| TEXAS INSTRUMENTS INCORPORATED
| Standard Linear and Logic Group
| IBIS Model of SN74AVCH16T245
| 16-Bit Dual-Supply Bus Transeiver with Configurable Voltage Translation and
| 3-State Outputs
| This file contains package information for the following:
|  TSSOP 48-pin (DGG) package as [Component] AVCH16T245_DGG
|  TVSOP 48-pin (DGV) package as [Component] AVCH16T245_DGV
|  U*BGA 48-pin (GQL) package as [Component] AVCH16T245_GQL
|  U*BGA 48-pin (ZQL) package as [Component] AVCH16T245_ZQL
| This device can be powered at the following Vccs:
|  1.2 volt Vcc
|  1.5 volt Vcc
|  1.8 volt Vcc
|  2.5 volt Vcc
|  3.3 volt Vcc
| This file provides unique models under the [Model Selector] for each Vcc.
| For operation at a specific Vcc, select the appropriate model after each
| [Model Selector] keyword.
[IBIS Ver]   3.2
[Comment char]  |_char
[File Name]   sn74avch16t245.ibs
[File Rev]   1.1 | x_die
[Date]   May 14, 2004
[Source]   Data created from TI-SPICE simulations at TI-SLL.
[Notes]   The following is an IBIS list for the AVCH16T245.
   Please contact sllibis@ti.com with questions and
   comments concerning SLL IBIS models.
   - FILE REV HISTORY
   - 1.1 Release IBIS file on 06/03/04
   - Power clamp data deleted as there is no power-clamp diode.
   - Non-monotonic data in ground-clamp due to bus-hold
   - Due to the fact that the Device is 4.6-V Input/Output
   tolarent, the I/O models has some Non-Monotonic Warnings.
[Disclaimer] Property of Texas Instruments Incorporated.  Unauthorized
   reproduction and/or distribution is strictly prohibited.
   This product is protected under copyright law.
   Created  2003, (C) Copyright  2003, Texas Instruments
   Incorporated, All Rights Reserved
   UNLESS THERE IS A SIGNED, WRITTEN AGREEMENT TO THE
   CONTRARY, TEXAS INSTRUMENTS (TI) IS PROVIDING THE IBIS
   MODELS  AND WITHOUT ANY WARRANTY, EXPRESSED OR
   IMPLIED.  TI assumes no liability for:
   1) the accuracy of the IBIS models provided to your
   company;
   2) the proper functioning of these IBIS Models in your
   design or for any resulting applications; or
   3) infringement of patents, copyrights or intellectual
   property rights resulting from your use of these IBIS
   models.
   TI provides IBIS Models as a service to our customers.
   You and your company shall not distribute, sell or give
   these models to anyone else without prior written
   permission from TI.
   TI reserves the right to make changes to our products or
   to discontinue any semiconductor product or service
   without notice, and advises our customers to obtain the
   latest version of relevant information to verify, before
   placing orders, that the information being relied on is
   current.
   Please be aware that your receipt and use of the IBIS
   information provided shall serve as acceptance of these
   terms and conditions.  If you do not accept these terms,
   you should return or destroy the IBIS models and any
   other accompanying information immediately.
| Component AVCH16T245_DGG 48-pin TSSOP
[Component]   AVCH16T245_DGG
[Manufacturer]   Texas Instruments, Inc.
[Package]
|   typ   min   max
R_pkg   6.200e-02   5.000e-02   7.800e-02
L_pkg   3.527e-09   3.128e-09   4.255e-09
C_pkg   5.300e-13   4.170e-13   6.850e-13
[Pin]   signal_name   model_name   R_pin   L_pin   C_pin
1   1DIR   AVCH16T245_DIR   5.000e-02   4.250e-09   6.710e-13
2   1b1   AVCH16T245_IO   5.700e-02   3.956e-09   6.740e-13
3   1b2   AVCH16T245_IO   7.100e-02   3.922e-09   6.190e-13
4   GND   GND   7.800e-02   3.841e-09   6.180e-13
5   1b3   AVCH16T245_IO   5.600e-02   3.535e-09   5.550e-13
6   1b4   AVCH16T245_IO   5.800e-02   3.464e-09   5.030e-13
7   VCCB   POWER   6.000e-02   3.362e-09   4.980e-13
8   1b5   AVCH16T245_IO   6.100e-02   3.293e-09   4.620e-13
9   1b6   AVCH16T245_IO   6.300e-02   3.240e-09   4.550e-13
10   GND   GND   6.300e-02   3.175e-09   4.420e-13
11   1b7   AVCH16T245_IO   6.400e-02   3.153e-09   4.290e-13
12   1b8   AVCH16T245_IO   6.500e-02   3.128e-09   4.180e-13
13   2b1   AVCH16T245_IO   6.500e-02   3.128e-09   4.180e-13
14   2b2   AVCH16T245_IO   6.400e-02   3.154e-09   4.290e-13
15   GND   GND   6.300e-02   3.174e-09   4.420e-13
16   2b3   AVCH16T245_IO   6.300e-02   3.241e-09   4.550e-13
17   2b4   AVCH16T245_IO   6.100e-02   3.293e-09   4.620e-13
18   VCCB   POWER   6.000e-02   3.362e-09   4.970e-13
19   2b5   AVCH16T245_IO   5.800e-02   3.464e-09   5.030e-13
20   2b6   AVCH16T245_IO   5.600e-02   3.537e-09   5.600e-13
21   GND   GND   7.700e-02   3.839e-09   6.260e-13
22   2b7   AVCH16T245_IO   7.100e-02   3.917e-09   6.270e-13
23   2b8   AVCH16T245_IO   5.800e-02   3.955e-09   6.850e-13
24   2dir   AVCH16T245_DIR   5.200e-02   4.255e-09   6.790e-13
25   2noe   AVCH16T245_NOE   5.100e-02   4.254e-09   6.760e-13
26   2a8   AVCH16T245_IO   5.800e-02   3.957e-09   6.790e-13
27   2a7   AVCH16T245_IO   7.100e-02   3.920e-09   6.210e-13
28   GND   GND   7.800e-02   3.843e-09   6.220e-13
29   2a6   AVCH16T245_IO   5.600e-02   3.539e-09   5.600e-13
30   2a5   AVCH16T245_IO   5.800e-02   3.466e-09   5.030e-13
31   VCCA   POWER   6.000e-02   3.363e-09   4.970e-13
32   2a4   AVCH16T245_IO   6.100e-02   3.294e-09   4.620e-13
33   2a3   AVCH16T245_IO   6.300e-02   3.241e-09   4.540e-13
34   GND   GND   6.300e-02   3.175e-09   4.410e-13
35   2a2   AVCH16T245_IO   6.400e-02   3.153e-09   4.290e-13
36   2a1   AVCH16T245_IO   6.500e-02   3.129e-09   4.170e-13
37   1a8   AVCH16T245_IO   6.500e-02   3.129e-09   4.170e-13
38   1a7   AVCH16T245_IO   6.400e-02   3.152e-09   4.290e-13
39   GND   GND   6.400e-02   3.176e-09   4.410e-13
40   1a6   AVCH16T245_IO   6.300e-02   3.241e-09   4.540e-13
41   1a5   AVCH16T245_IO   6.100e-02   3.293e-09   4.620e-13
42   VCCA   POWER   6.000e-02   3.363e-09   4.970e-13
43   1a4   AVCH16T245_IO   5.800e-02   3.464e-09   5.030e-13
44   1a3   AVCH16T245_IO   5.600e-02   3.534e-09   5.610e-13
45   GND   GND   7.800e-02   3.841e-09   6.260e-13
46   1a2   AVCH16T245_IO   7.100e-02   3.920e-09   6.220e-13
47   1a1   AVCH16T245_IO   5.700e-02   3.955e-09   6.770e-13
48   1noe   AVCH16T245_NOE   5.100e-02   4.252e-09   6.720e-13
| Component AVCH16T245_DGV 48-pin TVSOP
[Component]   AVCH16T245_DGV
[Manufacturer] Texas Instruments, Inc.
[Package]
|   typ   min   max
R_pkg   7.000e-02   4.900e-02   8.500e-02
L_pkg   3.013e-09   2.743e-09   3.408e-09
C_pkg   3.710e-13   2.940e-13   5.110e-13
[Pin]   signal_name   model_name   R_pin   L_pin   C_pin
1   1DIR   AVCH16T245_DIR   4.900e-02   3.393e-09   4.970e-13
2   1B1   AVCH16T245_IO   6.000e-02   3.250e-09   5.020e-13
3   1B2   AVCH16T245_IO   7.700e-02   3.310e-09   4.510e-13
4   GND   GND   8.500e-02   3.299e-09   4.040e-13
5   1B3   AVCH16T245_IO   8.300e-02   3.136e-09   3.600e-13
6   1B4   AVCH16T245_IO   7.700e-02   3.019e-09   3.630e-13
7   VCCB   POWER   6.500e-02   2.882e-09   3.490e-13
8   1B5   AVCH16T245_IO   6.600e-02   2.829e-09   3.140e-13
9   1B6   AVCH16T245_IO   6.700e-02   2.796e-09   3.140e-13
10   GND   GND   6.900e-02   2.754e-09   3.080e-13
11   1B7   AVCH16T245_IO   7.000e-02   2.753e-09   3.010e-13
12   1B8   AVCH16T245_IO   7.100e-02   2.745e-09   2.940e-13
13   2B1   AVCH16T245_IO   7.000e-02   2.744e-09   2.940e-13
14   2B2   AVCH16T245_IO   7.000e-02   2.754e-09   3.010e-13
15   GND   GND   6.900e-02   2.754e-09   3.080e-13
16   2B3   AVCH16T245_IO   6.700e-02   2.796e-09   3.140e-13
17   2B4   AVCH16T245_IO   6.600e-02   2.829e-09   3.140e-13
18   VCCB   POWER   6.500e-02   2.883e-09   3.500e-13
19   2B5   AVCH16T245_IO   7.500e-02   3.014e-09   3.630e-13
20   2B6   AVCH16T245_IO   8.000e-02   3.128e-09   3.580e-13
21   GND   GND   8.400e-02   3.295e-09   4.030e-13
22   2B7   AVCH16T245_IO   7.800e-02   3.311e-09   4.520e-13
23   2B8   AVCH16T245_IO   6.200e-02   3.259e-09   5.010e-13
24   2DIR   AVCH16T245_DIR   5.200e-02   3.404e-09   4.960e-13
25   2NOE   AVCH16T245_NOE   5.300e-02   3.397e-09   5.050e-13
26   2A8   AVCH16T245_IO   6.200e-02   3.249e-09   5.110e-13
27   2A7   AVCH16T245_IO   7.700e-02   3.308e-09   4.530e-13
28   GND   GND   8.200e-02   3.289e-09   4.030e-13
29   2A6   AVCH16T245_IO   7.800e-02   3.121e-09   3.590e-13
30   2A5   AVCH16T245_IO   7.400e-02   3.010e-09   3.630e-13
31   VCCA   POWER   6.500e-02   2.883e-09   3.490e-13
32   2A4   AVCH16T245_IO   6.700e-02   2.829e-09   3.140e-13
33   2A3   AVCH16T245_IO   6.700e-02   2.795e-09   3.140e-13
34   GND   GND   6.900e-02   2.753e-09   3.070e-13
35   2A2   AVCH16T245_IO   7.000e-02   2.753e-09   3.010e-13
36   2A1   AVCH16T245_IO   7.000e-02   2.743e-09   2.940e-13
37   1A8   AVCH16T245_IO   7.000e-02   2.743e-09   2.940e-13
38   1A7   AVCH16T245_IO   7.000e-02   2.753e-09   3.010e-13
39   GND   GND   6.900e-02   2.754e-09   3.070e-13
40   1A6   AVCH16T245_IO   6.800e-02   2.797e-09   3.140e-13
41   1A5   AVCH16T245_IO   6.700e-02   2.830e-09   3.140e-13
42   VCCA   POWER   6.400e-02   2.880e-09   3.490e-13
43   1A4   AVCH16T245_IO   7.200e-02   3.004e-09   3.620e-13
44   1A3   AVCH16T245_IO   7.800e-02   3.121e-09   3.590e-13
45   GND   GND   8.400e-02   3.296e-09   4.030e-13
46   1A2   AVCH16T245_IO   7.700e-02   3.308e-09   4.510e-13
47   1A1   AVCH16T245_IO   6.200e-02   3.258e-09   4.990e-13
48   1NOE   AVCH16T245_NOE   5.300e-02   3.408e-09   4.940e-13
| Component AVCH16T245_GQL 48-pin U*BGA
[Component]   AVCH16T245_GQL
[Manufacturer]   Texas Instruments, Inc.
[Package]
|   typ   min   max
R_pkg   7.900e-02   4.500e-02   9.400e-02
L_pkg   2.264e-09   1.398e-09   2.722e-09
C_pkg   3.060e-13   1.170e-13   4.040e-13
[Pin]   signal_name   model_name   R_pin   L_pin   C_pin
A1   1DIR   AVCH16T245_DIR   5.100e-02   1.531e-09   2.100e-13
B2   1B1   AVCH16T245_IO   7.300e-02   2.572e-09   3.120e-13
B1   1B2   AVCH16T245_IO   7.100e-02   1.835e-09   2.320e-13
B3   GND   GND   9.400e-02   2.717e-09   3.830e-13
C2   1B3   AVCH16T245_IO   8.900e-02   2.534e-09   3.500e-13
C1   1B4   AVCH16T245_IO   7.100e-02   1.831e-09   2.310e-13
C3   VCCB   POWER   9.400e-02   2.722e-09   3.920e-13
D2   1B5   AVCH16T245_IO   9.000e-02   2.551e-09   3.520e-13
D1   1B6   AVCH16T245_IO   7.200e-02   1.846e-09   2.440e-13
D3   GND   GND   9.400e-02   2.719e-09   4.030e-13
E2   1B7   AVCH16T245_IO   8.900e-02   2.541e-09   3.510e-13
E1   1B8   AVCH16T245_IO   7.200e-02   1.850e-09   2.270e-13
F1   2B1   AVCH16T245_IO   7.200e-02   1.850e-09   2.270e-13
F2   2B2   AVCH16T245_IO   8.900e-02   2.541e-09   3.510e-13
G3   GND   GND   9.400e-02   2.718e-09   4.040e-13
G1   2B3   AVCH16T245_IO   7.200e-02   1.847e-09   2.440e-13
G2   2B4   AVCH16T245_IO   9.000e-02   2.551e-09   3.520e-13
H3   VCCB   POWER   9.400e-02   2.721e-09   3.920e-13
H1   2B5   AVCH16T245_IO   7.000e-02   1.830e-09   2.310e-13
H2   2B6   AVCH16T245_IO   8.800e-02   2.524e-09   3.500e-13
J3   GND   GND   9.300e-02   2.709e-09   3.820e-13
J1   2B7   AVCH16T245_IO   7.100e-02   1.851e-09   2.330e-13
J2   2B8   AVCH16T245_IO   5.600e-02   2.605e-09   3.900e-13
K1   2DIR   AVCH16T245_DIR   4.500e-02   1.398e-09   1.170e-13
K6   2NOE   AVCH16T245_NOE   4.500e-02   1.512e-09   1.930e-13
J5   2A8   AVCH16T245_IO   5.500e-02   2.492e-09   3.130e-13
J6   2A7   AVCH16T245_IO   7.000e-02   1.821e-09   2.300e-13
J4   GND   GND   9.300e-02   2.703e-09   3.820e-13
H5   2A6   AVCH16T245_IO   8.900e-02   2.529e-09   3.500e-13
H6   2A5   AVCH16T245_IO   7.100e-02   1.826e-09   2.300e-13
H4   VCCA   POWER   9.400e-02   2.722e-09   3.910e-13
G5   2A4   AVCH16T245_IO   9.000e-02   2.551e-09   3.520e-13
G6   2A3   AVCH16T245_IO   7.200e-02   1.846e-09   2.440e-13
G4   GND   GND   9.400e-02   2.719e-09   4.040e-13
F5   2A2   AVCH16T245_IO   8.800e-02   2.510e-09   3.490e-13
F6   2A1   AVCH16T245_IO   7.200e-02   1.850e-09   2.270e-13
E6   1A8   AVCH16T245_IO   7.100e-02   1.850e-09   2.270e-13
E5   1A7   AVCH16T245_IO   8.900e-02   2.529e-09   3.500e-13
D4   GND   GND   9.400e-02   2.719e-09   4.030e-13
D6   1A6   AVCH16T245_IO   7.200e-02   1.847e-09   2.430e-13
D5   1A5   AVCH16T245_IO   8.900e-02   2.550e-09   3.520e-13
C4   VCCA   POWER   9.400e-02   2.722e-09   3.910e-13
C6   1A4   AVCH16T245_IO   7.100e-02   1.827e-09   2.300e-13
C5   1A3   AVCH16T245_IO   8.900e-02   2.539e-09   3.500e-13
B4   GND   GND   9.300e-02   2.705e-09   3.820e-13
B6   1A2   AVCH16T245_IO   7.100e-02   1.831e-09   2.270e-13
B5   1A1   AVCH16T245_IO   7.300e-02   2.685e-09   3.800e-13
A6   1NOE   AVCH16T245_NOE   5.100e-02   1.417e-09   1.330e-13
| Component AVCH16T245_ZQL 48-pin U*BGA
[Component]   AVCH16T245_ZQL
[Manufacturer]   Texas Instruments, Inc.
[Package]
|   typ   min   max
R_pkg   7.900e-02   4.500e-02   9.400e-02
L_pkg   2.264e-09   1.398e-09   2.722e-09
C_pkg   3.060e-13   1.170e-13   4.040e-13
[Pin]   signal_name   model_name   R_pin   L_pin   C_pin
A1   1DIR   AVCH16T245_DIR   5.100e-02   1.531e-09   2.100e-13
B2   1B1   AVCH16T245_IO   7.300e-02   2.572e-09   3.120e-13
B1   1B2   AVCH16T245_IO   7.100e-02   1.835e-09   2.320e-13
B3   GND   GND   9.400e-02   2.717e-09   3.830e-13
C2   1B3   AVCH16T245_IO   8.900e-02   2.534e-09   3.500e-13
C1   1B4   AVCH16T245_IO   7.100e-02   1.831e-09   2.310e-13
C3   VCCB   POWER   9.400e-02   2.722e-09   3.920e-13
D2   1B5   AVCH16T245_IO   9.000e-02   2.551e-09   3.520e-13
D1   1B6   AVCH16T245_IO   7.200e-02   1.846e-09   2.440e-13
D3   GND   GND   9.400e-02   2.719e-09   4.030e-13
E2   1B7   AVCH16T245_IO   8.900e-02   2.541e-09   3.510e-13
E1   1B8   AVCH16T245_IO   7.200e-02   1.850e-09   2.270e-13
F1   2B1   AVCH16T245_IO   7.200e-02   1.850e-09   2.270e-13
F2   2B2   AVCH16T245_IO   8.900e-02   2.541e-09   3.510e-13
G3   GND   GND   9.400e-02   2.718e-09   4.040e-13
G1   2B3   AVCH16T245_IO   7.200e-02   1.847e-09   2.440e-13
G2   2B4   AVCH16T245_IO   9.000e-02   2.551e-09   3.520e-13
H3   VCCB   POWER   9.400e-02   2.721e-09   3.920e-13
H1   2B5   AVCH16T245_IO   7.000e-02   1.830e-09   2.310e-13
H2   2B6   AVCH16T245_IO   8.800e-02   2.524e-09   3.500e-13
J3   GND   GND   9.300e-02   2.709e-09   3.820e-13
J1   2B7   AVCH16T245_IO   7.100e-02   1.851e-09   2.330e-13
J2   2B8   AVCH16T245_IO   5.600e-02   2.605e-09   3.900e-13
K1   2DIR   AVCH16T245_DIR   4.500e-02   1.398e-09   1.170e-13
K6   2NOE   AVCH16T245_NOE   4.500e-02   1.512e-09   1.930e-13
J5   2A8   AVCH16T245_IO   5.500e-02   2.492e-09   3.130e-13
J6   2A7   AVCH16T245_IO   7.000e-02   1.821e-09   2.300e-13
J4   GND   GND   9.300e-02   2.703e-09   3.820e-13
H5   2A6   AVCH16T245_IO   8.900e-02   2.529e-09   3.500e-13
H6   2A5   AVCH16T245_IO   7.100e-02   1.826e-09   2.300e-13
H4   VCCA   POWER   9.400e-02   2.722e-09   3.910e-13
G5   2A4   AVCH16T245_IO   9.000e-02   2.551e-09   3.520e-13
G6   2A3   AVCH16T245_IO   7.200e-02   1.846e-09   2.440e-13
G4   GND   GND   9.400e-02   2.719e-09   4.040e-13
F5   2A2   AVCH16T245_IO   8.800e-02   2.510e-09   3.490e-13
F6   2A1   AVCH16T245_IO   7.200e-02   1.850e-09   2.270e-13
E6   1A8   AVCH16T245_IO   7.100e-02   1.850e-09   2.270e-13
E5   1A7   AVCH16T245_IO   8.900e-02   2.529e-09   3.500e-13
D4   GND   GND   9.400e-02   2.719e-09   4.030e-13
D6   1A6   AVCH16T245_IO   7.200e-02   1.847e-09   2.430e-13
D5   1A5   AVCH16T245_IO   8.900e-02   2.550e-09   3.520e-13
C4   VCCA   POWER   9.400e-02   2.722e-09   3.910e-13
C6   1A4   AVCH16T245_IO   7.100e-02   1.827e-09   2.300e-13
C5   1A3   AVCH16T245_IO   8.900e-02   2.539e-09   3.500e-13
B4   GND   GND   9.300e-02   2.705e-09   3.820e-13
B6   1A2   AVCH16T245_IO   7.100e-02   1.831e-09   2.270e-13
B5   1A1   AVCH16T245_IO   7.300e-02   2.685e-09   3.800e-13
A6   1NOE   AVCH16T245_NOE   5.100e-02   1.417e-09   1.330e-13
| Model AVCH16T245_DIR
[Model Selector]   AVCH16T245_DIR
AVCH16T245_DIR_12   1.2 volt Vcc
AVCH16T245_DIR_15   1.5 volt Vcc
AVCH16T245_DIR_18   1.8 volt Vcc
AVCH16T245_DIR_25   2.5 volt Vcc
AVCH16T245_DIR_33   3.3 volt Vcc
| Model AVCH16T245_NOE
[Model Selector]   AVCH16T245_NOE
AVCH16T245_NOE_12   1.2 volt Vcc
AVCH16T245_NOE_15   1.5 volt Vcc
AVCH16T245_NOE_18   1.8 volt Vcc
AVCH16T245_NOE_25   2.5 volt Vcc
AVCH16T245_NOE_33   3.3 volt Vcc
| Model AVCH16T245_IO
[Model Selector]   AVCH16T245_IO
AVCH16T245_IO_12   1.2 volt Vcc
AVCH16T245_IO_15   1.5 volt Vcc
AVCH16T245_IO_18   1.8 volt Vcc
AVCH16T245_IO_25   2.5 volt Vcc
AVCH16T245_IO_33   3.3 volt Vcc
| Models and submodels in the file (15): AVCH16T245_DIR_12 (Input), AVCH16T245_DIR_15 (Input), AVCH16T245_DIR_18 (Input), AVCH16T245_DIR_25 (Input), AVCH16T245_DIR_33 (Input), AVCH16T245_NOE_12 (Input), AVCH16T245_NOE_15 (Input), AVCH16T245_NOE_18 (Input), AVCH16T245_NOE_25 (Input), AVCH16T245_NOE_33 (Input), AVCH16T245_IO_12 (I/O), AVCH16T245_IO_15 (I/O), AVCH16T245_IO_18 (I/O), AVCH16T245_IO_25 (I/O), AVCH16T245_IO_33 (I/O)
